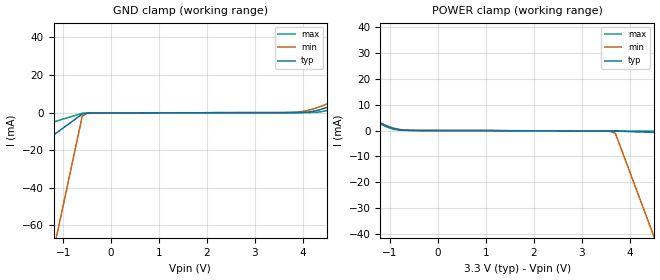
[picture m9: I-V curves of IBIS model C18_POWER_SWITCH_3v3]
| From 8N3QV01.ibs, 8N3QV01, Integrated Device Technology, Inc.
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[Model] C18_POWER_SWITCH_3v3
Model_type   Input
Polarity   Non-Inverting
Vinl = 0.8V
Vinh = 2.0V
|   typ   min   max
C_comp   2pF   1.5pF   2.5pF
|   typ   min   max
[Voltage range]   3.3V   3.135V   3.465V
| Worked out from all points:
|   GND clamp passes 1 mA (typ) near -0.61 V on its own axis
|   POWER clamp passes 1 mA (typ) near -0.97 V on its own axis
[GND_clamp]
|Voltage   I (typ)   I (min)   I (max)
-3.3V     -51.02mA   -323.8mA   -21.16mA
-1.2V     -11.9mA    -73.33mA   -4.953mA
-1.1V     -10.04mA   -61.41mA   -4.181mA
-600mV    -721.5uA   -1.785mA   -323.1uA
-500mV    -290.1uA   -488.1uA   -210.5uA
3.8V      30.67uA    140.9uA    5.709uA
4.2V      626.5uA    1.86mA     95.33uA
4.5V      2.802mA    4.615mA    1.157mA
4.9V      7.755mA    9.775mA    5.675mA
5.3V      14.54mA    16.34mA    12.83mA
5.7V      22.76mA    24.05mA    21.93mA
6.6V      43.51mA    43.11mA    45.31mA
[Power_clamp]
|Voltage   I (typ)   I (min)   I (max)
-3.3V     42.96mA    38.61mA    50.07mA
-3.2V     40.72mA    36.62mA    47.41mA
-2.9V     33.98mA    30.67mA    39.43mA
-2.2V     18.49mA    16.97mA    21.07mA
-1.8V     10.95mA    10.3mA     12.12mA
-1.3V     3.842mA    3.929mA    3.813mA
-900mV    626.5uA    835.5uA    405.4uA
-400mV    10.84uA    21.25uA    6.941uA
3.6V      -216.8uA   -363.4uA   -183.6uA
3.7V      -227.6uA   -1.065mA   -189.3uA
4.5V      -727.6uA   -40.95mA   -234.8uA
6.6V      -2.04mA    -145.6mA   -354.2uA
